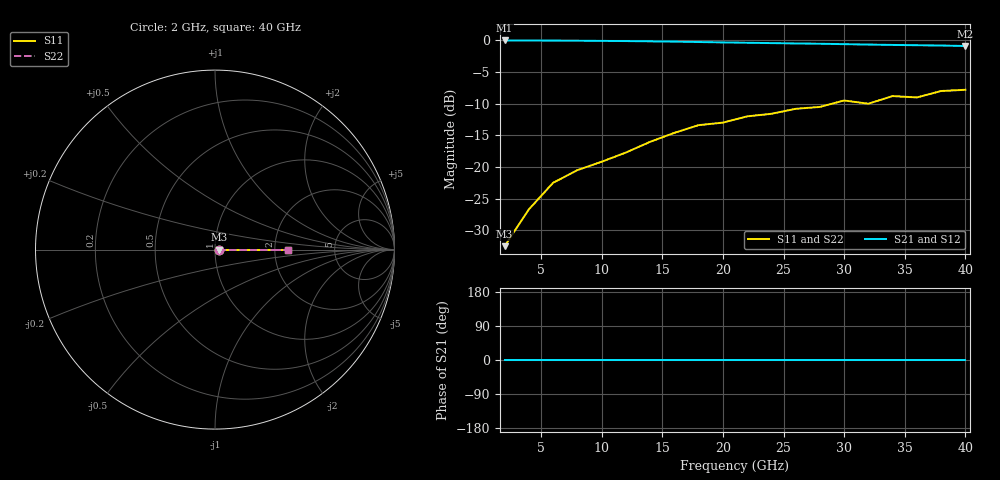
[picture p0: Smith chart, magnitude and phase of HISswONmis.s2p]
# GHZ S MA R 50
!Output file by Shape3_28
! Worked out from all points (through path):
!   20 points, 2 GHz to 40 GHz, reference 50 ohm
!   highest |S21| = -0.02 dB at 2 GHz (marker M1); lowest = -0.9 dB at 40 GHz (marker M2)
!   lowest |S11| = -32.5 dB at 2 GHz (marker M3), VSWR 1.05, Z = 52.4 + j0 ohm
!   |S11| at or under -10 dB: start of sweep to 29.01 GHz; 31.97532 GHz to 32.01039 GHz (35.07 MHz wide, 0.11 % of centre)
!   |S22| runs from -32.5 to -7.8 dB; largest |S21 - S12| = 0.0095
2  0.0237 0.0  0.9979 0.0  0.9979 0.0  0.0237 0.0
4  0.0463 0.0  0.9972 0.0  0.9972 0.0  0.0463 0.0
6  0.075 0.0  0.9951 0.0  0.9951 0.0  0.075 0.0
8  0.0944 0.0  0.9934 0.0  0.9934 0.0  0.0944 0.0
10  0.11 0.0  0.99 0.0  0.9917 0.0  0.11 0.0
12  0.13 0.0  0.987 0.0  0.9965 0.0  0.13 0.0
14  0.158 0.0  0.982 0.0  0.983 0.0  0.158 0.0
16  0.186 0.0  0.977 0.0  0.973 0.0  0.186 0.0
18  0.214 0.0  0.97 0.0  0.968 0.0  0.214 0.0
20  0.224 0.0  0.963 0.0  0.96 0.0  0.224 0.0
22  0.251 0.0  0.957 0.0  0.95 0.0  0.251 0.0
24  0.263 0.0  0.951 0.0  0.944 0.0  0.263 0.0
26  0.288 0.0  0.945 0.0  0.938 0.0  0.288 0.0
28  0.298 0.0  0.94 0.0  0.9332 0.0  0.298 0.0
30  0.335 0.0  0.933 0.0  0.9279 0.0  0.335 0.0
32  0.316 0.0  0.926 0.0  0.9225 0.0  0.316 0.0
34  0.363 0.0  0.92 0.0  0.917 0.0  0.363 0.0
36  0.354 0.0  0.915 0.0  0.912 0.0  0.354 0.0
38  0.398 0.0  0.91 0.0  0.906 0.0  0.398 0.0
40  0.407 0.0  0.902 0.0  0.902 0.0  0.407 0.0
